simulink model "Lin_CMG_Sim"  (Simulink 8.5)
settings: Solver=ode3  StartTime=0.0  StopTime=1000  FixedStep=Ts  RelTol=1e-3
InitFcn:
  | start
StopFcn:
  | Pl
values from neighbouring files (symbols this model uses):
  Ave = [    [vehicle_flex34.m]    (also in vehicle_rigid.m)
  Bve = [    [vehicle_flex34.m]    (also in vehicle_rigid.m)
  Cve = [    [vehicle_flex34.m]    (also in vehicle_rigid.m)
  d2r = pi/180    (= 0.0174532925199)    [Dead_Band_DF.m]    (also in start.m; start1.m; start2.m; start3.m)
  Dve = [    [vehicle_flex34.m]    (also in vehicle_rigid.m)
  J = [0.119416e9, -0.476e7,   -0.1216e7;     -0.476e7,     0.40408e8, -0.30121e6;     -0.1216e7,   -0.30121e6,  0.110166e9]    [start.m]    (also in start1.m; start2.m; start3.m)
  omg = 20*wo    (= 0.022)    [start.m]    (also in start1.m; start2.m; start3.m)
  r2d = 180/pi    (= 57.2957795131)    [start.m]    (also in start1.m; start2.m; start3.m)
  zeb = 0.95    [start.m]    (also in start1.m; start2.m; start3.m)
undefined symbols (not defined in the file or in its folder): Torq_Lim

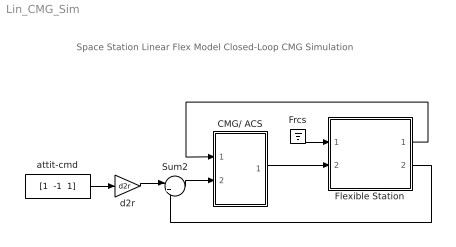
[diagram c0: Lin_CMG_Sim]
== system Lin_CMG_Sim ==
  note: Space Station Linear Flex Model Closed-Loop CMG Simulation
  CMG/ ACS : Subsystem
  Flexible Station : Subsystem
  Frcs : Ground
  Sum2 : Sum  Inputs=|+-
  attit-cmd : Constant  Value="[1  -1  1]"
  d2r : Gain  Gain=d2r
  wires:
  Flexible Station/1(wbf) -> CMG/ ACS/1(wb)
  attit-cmd/1 -> d2r/1
  d2r/1 -> Sum2/1
  Flexible Station/2(att) -> Sum2/2
  Frcs/1 -> Flexible Station/1(Frcs)
  CMG/ ACS/1(Tq) -> Flexible Station/2(Tcmg)
  Sum2/1 -> CMG/ ACS/2(ater)

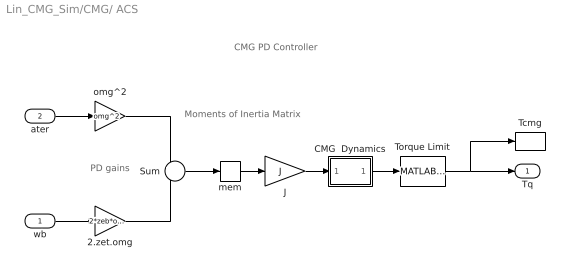
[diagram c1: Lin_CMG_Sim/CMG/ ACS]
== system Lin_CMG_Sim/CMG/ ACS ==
  note: CMG PD Controller
  note: PD gains
  note: Moments of Inertia Matrix
  wb : Inport
  ater : Inport  Port=2  PortDimensions=3
  2.zet.omg : Gain  Gain=2*zeb*omg
  CMG  Dynamics : Subsystem
  J : Gain  Gain=J  Multiplication=Matrix(K*u)
  Sum : Sum  Inputs=+-
  Tcmg : ToWorkspace  VariableName=Tcmg  SampleTime=-1
  Torque Limit : MATLABFcn  MATLABFcn=Torq_Lim( u(1:3) )  OutputDimensions=3
  mem : Memory
  omg^2 : Gain  Gain=omg^2
  Tq : Outport
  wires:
  wb/1 -> 2.zet.omg/1
  Sum/1 -> mem/1
  2.zet.omg/1 -> Sum/2
  ater/1 -> omg^2/1
  omg^2/1 -> Sum/1
  J/1 -> CMG  Dynamics/1(I)
  mem/1 -> J/1
  CMG  Dynamics/1(O) -> Torque Limit/1
  Torque Limit/1 -> Tq/1, Tcmg/1

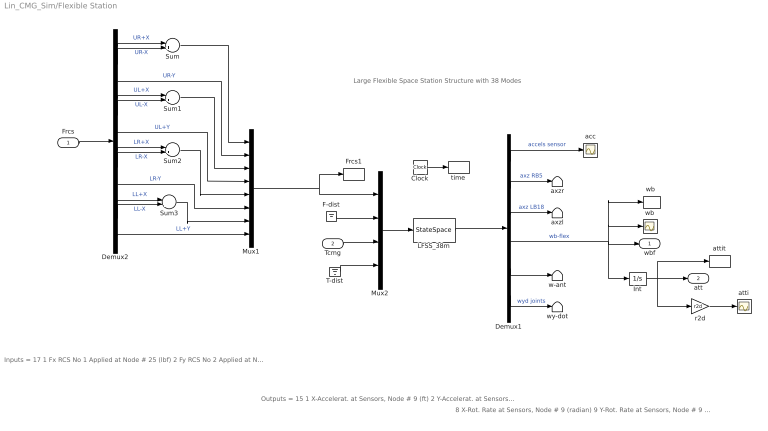
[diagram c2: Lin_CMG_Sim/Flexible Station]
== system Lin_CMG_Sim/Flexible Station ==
  note: Outputs = 15 1 X-Accelerat. at Sensors, Node # 9 (ft) 2 Y-Accelerat. at Sensors, Node # 9 (ft) 3 Z-Accelerat. at Sensors, Node # 9 (ft) 4 X-Accelerat. at Right Boom End, Node # 5 (ft) 5 Z-Accelerat. at Right Boom End, Node # 5 (ft) 6 X-Accelerat. at Left Boom End, Node # 18 (ft) 7 Z-Accelerat. at Left Boom End, Node # 18 (ft)
  note: Inputs = 17 1 Fx RCS No 1 Applied at Node # 25 (lbf) 2 Fy RCS No 2 Applied at Node # 25 (lbf) 3 Fx RCS No 3 Applied at Node # 26 (lbf) 4 Fy RCS No 4 Applied at Node # 26 (lbf) 5 Fx RCS No 5 Applied at Node # 27 (lbf) 6 Fy RCS No 6 Applied at Node # 27 (lbf) 7 Fx RCS No 7 Applied at Node # 28 (lbf) 8 Fy RCS No 8 Applied at Node # 28 (lbf) 9 Fx Disturb. No 9 at Node # 21 (lbf) 10 Fy Disturb. No 10 at Node # 21 (lbf) 11 Fz Disturb. No 11 at Node # 21 (lbf) 12 Torq-x No 1 CMG Applied at Node # 10 (ft-lb) 13 Torq-y No 2 CMG Applied at Node # 10 (ft-lb) 14 Torq-z No 3 CMG Applied at Node # 10 (ft-lb) 15 Torq-x No 4 Gimbal Dist. at Node # 1 (ft-lb) 16 Torq-y No 5 Gimbal Dist. at Node # 1 (ft-lb) 17 Torq-z No 6 Gimbal Dist. at Node # 1 (ft-lb)
  note: Large Flexible Space Station Structure with 38 Modes
  note: 8 X-Rot. Rate at Sensors, Node # 9 (radian) 9 Y-Rot. Rate at Sensors, Node # 9 (radian) 10 Z-Rot. Rate at Sensors, Node # 9 (radian) 11 X-Rot. Rate at Antena Bot-Left, Node # 24 (radian) 12 Y-Rot. Rate at Antena Bot-Left, Node # 24 (radian) 13 Z-Rot. Rate at Antena Bot-Left, Node # 24 (radian) 14 Y-Rot.Accel. at Right Joint, Node # 7 (radian) 15 Y-Rot.Accel. at Left Joint, Node # 16 (radian)
  Frcs : Inport
  Tcmg : Inport  Port=2
  Clock : Clock
  Demux1 : Demux  Outputs=[3, 2, 2, 3, 3, 2]
  Demux2 : Demux  Outputs=12
  F-dist : Ground
  Frcs1 : ToWorkspace  VariableName=Frcs  SampleTime=-1
  Int : Integrator
  LFSS_38m : StateSpace  A=Ave  B=Bve  C=Cve  D=Dve  X0=0
  Mux1 : Mux  Inputs=8
  Mux2 : Mux  Inputs=[8, 3, 3, 3]
  Sum{,1..3} (4 alike) : Sum  Inputs=|+-
  T-dist : Ground
  acc : Scope
  atti : Scope
  attit : ToWorkspace  VariableName=atti  SampleTime=-1
  axzl : Terminator
  axzr : Terminator
  r2d : Gain  Gain=r2d
  time : ToWorkspace  VariableName=time  SampleTime=-1
  w-ant : Terminator
  wb : Scope
  "wb " : ToWorkspace  VariableName=wb  SampleTime=-1
  wy-dot : Terminator
  wbf : Outport
  att : Outport  Port=2
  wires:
  Demux1/6 -> wy-dot/1  "wyd joints"
  Demux1/5 -> w-ant/1
  T-dist/1 -> Mux2/4
  F-dist/1 -> Mux2/2
  Demux1/3 -> axzl/1  "axz LB18"
  Demux1/2 -> axzr/1  "axz RB5"
  Tcmg/1 -> Mux2/3
  Demux1/4 -> wbf/1, Int/1, wb/1, "wb "/1  "wb-flex"
  Demux1/1 -> acc/1  "accels sensor"
  LFSS_38m/1 -> Demux1/1
  Clock/1 -> time/1
  Mux2/1 -> LFSS_38m/1
  Mux1/1 -> Mux2/1, Frcs1/1
  Frcs/1 -> Demux2/1
  Demux2/6 -> Mux1/4  "UL+Y"
  Demux2/9 -> Mux1/6  "LR-Y"
  Demux2/12 -> Mux1/8  "LL+Y"
  Demux2/3 -> Mux1/2  "UR-Y"
  Demux2/1 -> Sum/1  "UR+X"
  Demux2/2 -> Sum/2  "UR-X"
  Sum/1 -> Mux1/1
  Demux2/4 -> Sum1/1  "UL+X"
  Demux2/5 -> Sum1/2  "UL-X"
  Sum1/1 -> Mux1/3
  Demux2/7 -> Sum2/1  "LR+X"
  Demux2/8 -> Sum2/2  "LR-X"
  Demux2/10 -> Sum3/1  "LL+X"
  Demux2/11 -> Sum3/2  "LL-X"
  Sum3/1 -> Mux1/7
  Sum2/1 -> Mux1/5
  r2d/1 -> atti/1
  Int/1 -> att/1, r2d/1, attit/1

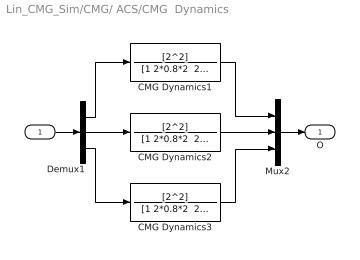
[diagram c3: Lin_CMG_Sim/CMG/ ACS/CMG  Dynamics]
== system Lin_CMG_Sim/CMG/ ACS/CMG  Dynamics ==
  I : Inport
  CMG Dynamics1 : TransferFcn  Numerator=[2^2]  Denominator="[1 2*0.8*2  2^2]"
  CMG Dynamics2 : TransferFcn  Numerator=[2^2]  Denominator="[1 2*0.8*2  2^2]"
  CMG Dynamics3 : TransferFcn  Numerator=[2^2]  Denominator="[1 2*0.8*2  2^2]"
  Demux1 : Demux  Outputs=3
  Mux2 : Mux  Inputs=3
  O : Outport
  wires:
  CMG Dynamics2/1 -> Mux2/2
  CMG Dynamics3/1 -> Mux2/3
  CMG Dynamics1/1 -> Mux2/1
  Demux1/2 -> CMG Dynamics2/1
  Demux1/1 -> CMG Dynamics1/1
  Demux1/3 -> CMG Dynamics3/1
  I/1 -> Demux1/1
  Mux2/1 -> O/1
